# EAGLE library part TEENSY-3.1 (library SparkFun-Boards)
Teensy 3+ Footprint Mechanical footprint with connectors for Teensy Development Board with ARM Cortex. SparkFun Products: Teensy 3.2 Teensy LC
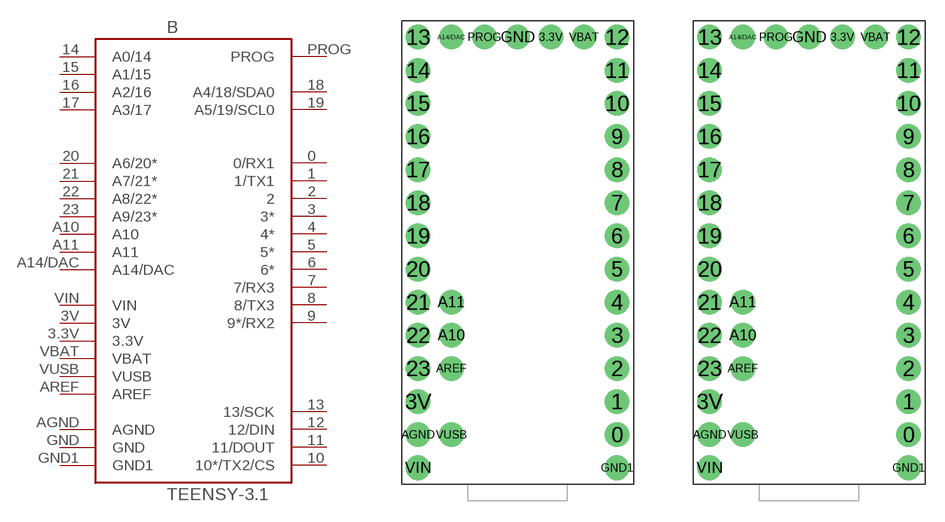
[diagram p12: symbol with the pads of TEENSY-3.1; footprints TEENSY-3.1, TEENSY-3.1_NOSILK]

Designator prefix B

## TEENSY-3.1SILK (SF_ID: DEV-12646)  [TEENSY-3.1]
0  0/RX1
1  1/TX1
2  2
3  3*
3.3V  3.3V
3V  3V
4  4*
5  5*
6  6*
7  7/RX3
8  8/TX3
9  9*/RX2
10  10*/TX2/CS
11  11/DOUT
12  12/DIN
13  13/SCK
14  A0/14
15  A1/15
16  A2/16
17  A3/17
18  A4/18/SDA0
19  A5/19/SCL0
20  A6/20*
21  A7/21*
22  A8/22*
23  A9/23*
A10  A10
A11  A11
A14/DAC  A14/DAC
AGND  AGND
AREF  AREF
GND  GND
GND1  GND1
PROG  PROG
VBAT  VBAT
VIN  VIN
VUSB  VUSB

## TEENSY-3.1NOSILK (SF_ID: DEV-12646)  [TEENSY-3.1_NOSILK]
Pads as for TEENSY-3.1

## Footprint TEENSY-3.1 (pad centres in mm)
drill 1.016 pad 1.88: 0 16.51,3.81; 1 16.51,6.35; 2 16.51,8.89; 3 16.51,11.43; 3.3V 11.43,34.29; 3V 1.27,6.35; 4 16.51,13.97; 5 16.51,16.51; 6 16.51,19.05; 7 16.51,21.59; 8 16.51,24.13; 9 16.51,26.67; 10 16.51,29.21; 11 16.51,31.75; 12 16.51,34.29; 13 1.27,34.29; 14 1.27,31.75; 15 1.27,29.21; 16 1.27,26.67; 17 1.27,24.13; 18 1.27,21.59; 19 1.27,19.05; 20 1.27,16.51; 21 1.27,13.97; 22 1.27,11.43; 23 1.27,8.89; A10 3.81,11.43; A11 3.81,13.97; A14/DAC 3.81,34.29; AGND 1.27,3.81; AREF 3.81,8.89; GND 8.89,34.29; GND1 16.51,1.27; PROG 6.35,34.29; VBAT 13.97,34.29; VIN 1.27,1.27; VUSB 3.81,3.81

## Footprint TEENSY-3.1_NOSILK (pad centres in mm)
drill 1.016 pad 1.88: 0 16.51,3.81; 1 16.51,6.35; 2 16.51,8.89; 3 16.51,11.43; 3.3V 11.43,34.29; 3V 1.27,6.35; 4 16.51,13.97; 5 16.51,16.51; 6 16.51,19.05; 7 16.51,21.59; 8 16.51,24.13; 9 16.51,26.67; 10 16.51,29.21; 11 16.51,31.75; 12 16.51,34.29; 13 1.27,34.29; 14 1.27,31.75; 15 1.27,29.21; 16 1.27,26.67; 17 1.27,24.13; 18 1.27,21.59; 19 1.27,19.05; 20 1.27,16.51; 21 1.27,13.97; 22 1.27,11.43; 23 1.27,8.89; A10 3.81,11.43; A11 3.81,13.97; A14/DAC 3.81,34.29; AGND 1.27,3.81; AREF 3.81,8.89; GND 8.89,34.29; GND1 16.51,1.27; PROG 6.35,34.29; VBAT 13.97,34.29; VIN 1.27,1.27; VUSB 3.81,3.81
